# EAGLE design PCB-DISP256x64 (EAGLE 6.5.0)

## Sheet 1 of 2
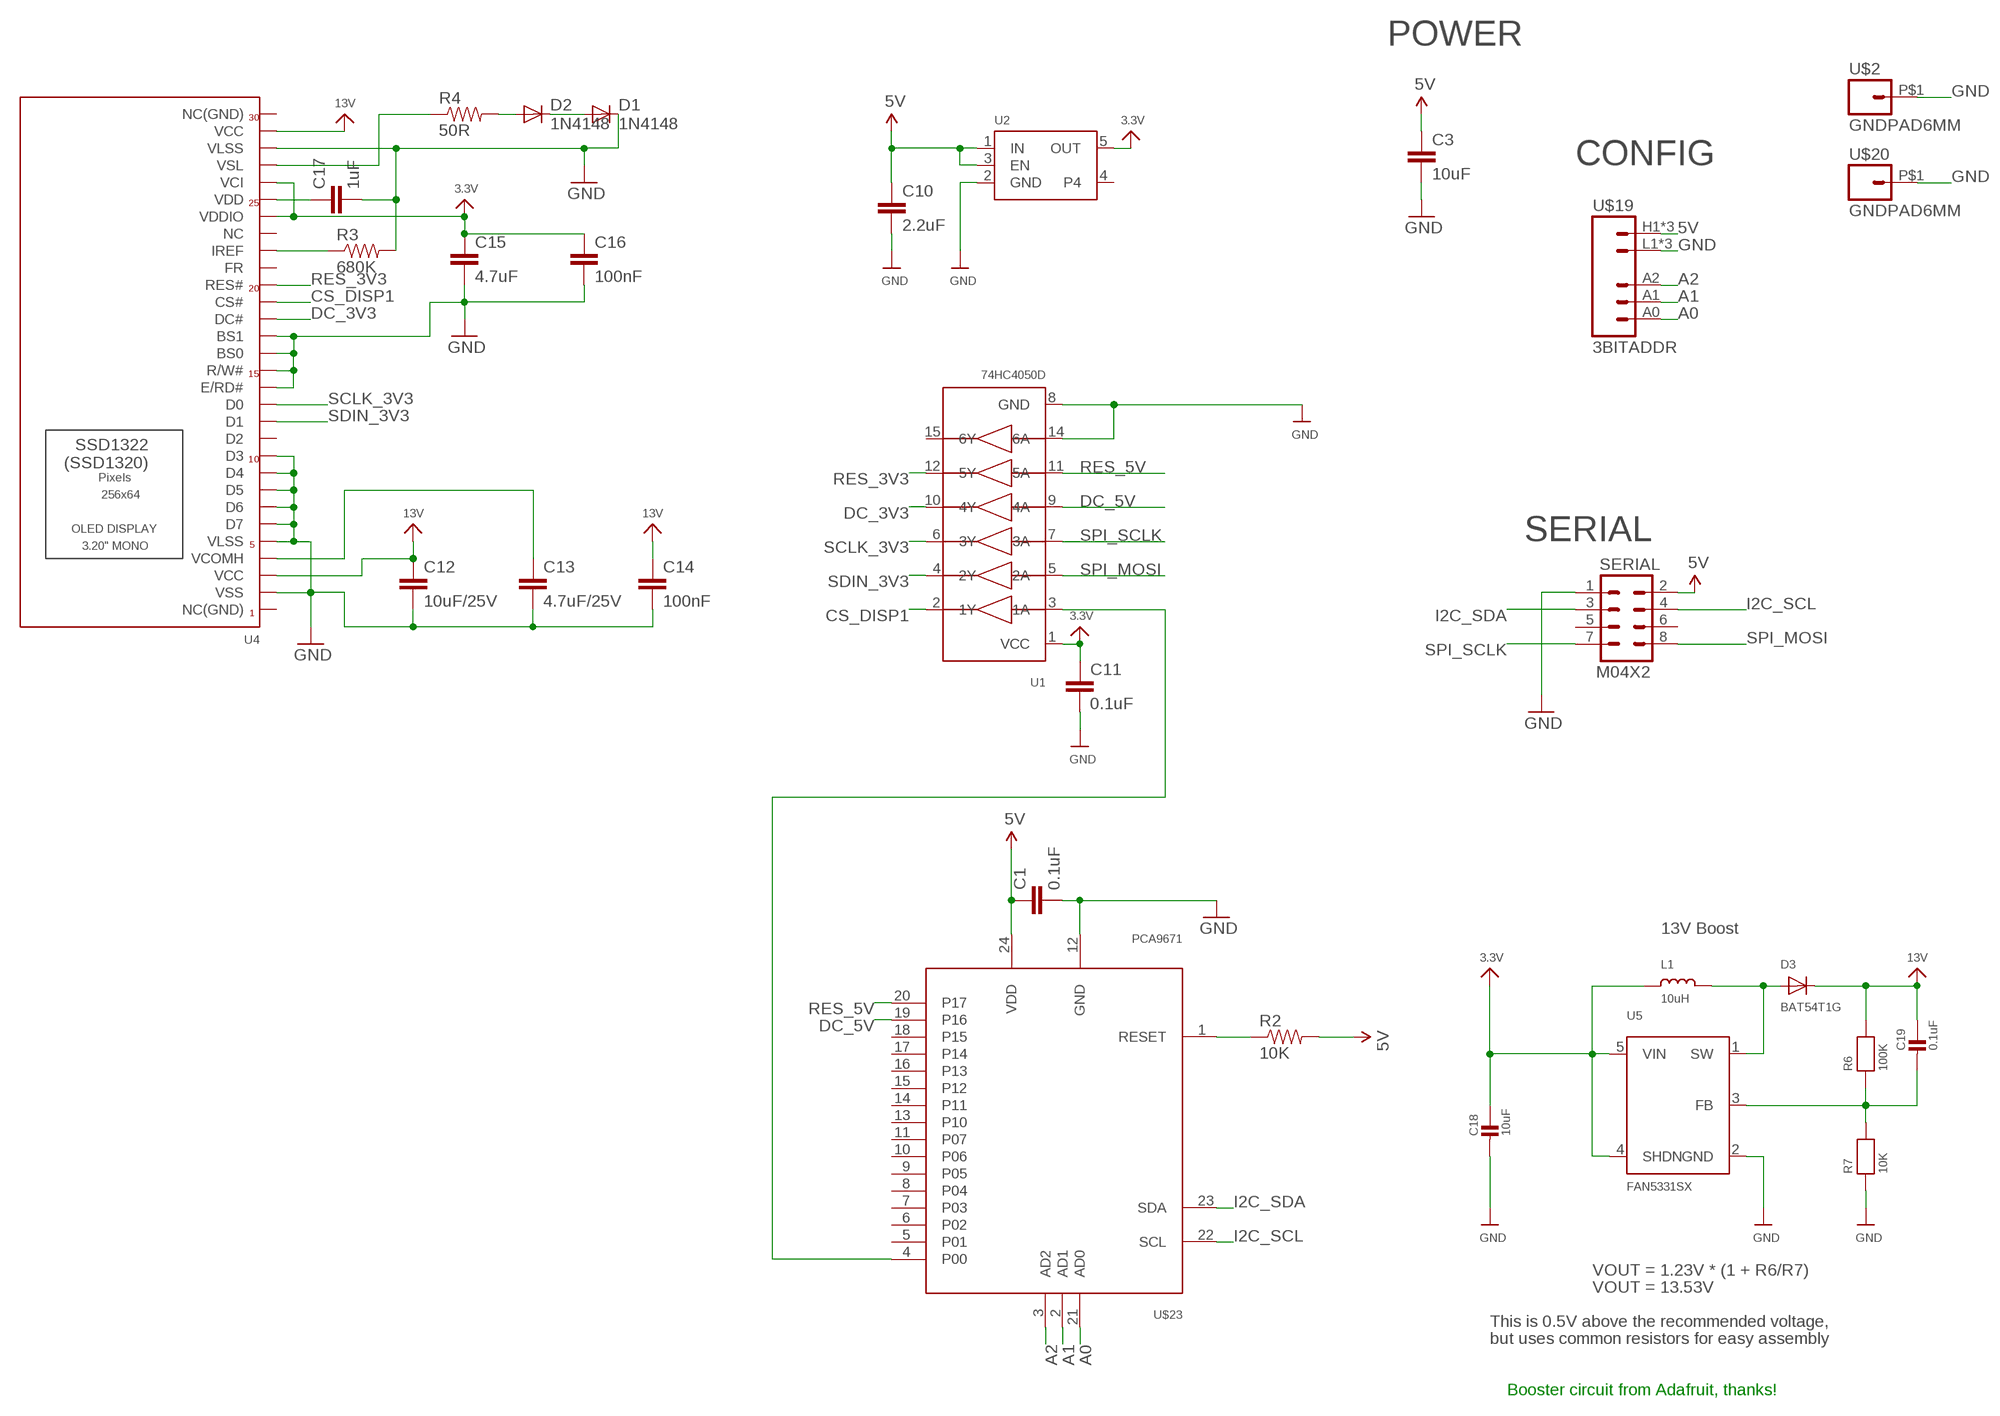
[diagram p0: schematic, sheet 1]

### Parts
C1  0.1uF  CAP0603-CAP  [0603-CAP]
C3  10uF  CAP0805  [0805]
C10  2.2uF  CAP0603-CAP  [0603-CAP]
C11  0.1uF  CAP0603-CAP  [0603-CAP]
C12  10uF/25V  CAP0805  [0805]
C13  4.7uF/25V  CAP0805  [0805]
C14  100nF  CAP0603-CAP  [0603-CAP]
C15  4.7uF  CAP0805  [0805]
C16  100nF  CAP0603-CAP  [0603-CAP]
C17  1uF  CAP0603-CAP  [0603-CAP]
C18  10uF  CAP_CERAMIC0805  [0805]
C19  0.1uF  CAP_CERAMIC0805  [0805]
D1  1N4148  DIODESOD  [SOD-323]
D2  1N4148  DIODESOD  [SOD-323]
D3  BAT54T1G  DIODESOD-123  [SOD-123]
L1  10uH  INDUCTOR  [INDUCTOR_1007]
R2  10K  RESISTOR0603-RES  [0603-RES]
R3  680K  RESISTOR0603-RES  [0603-RES]
R4  50R  RESISTOR0603-RES  [0603-RES]
R6  100K  RESISTOR0805  [0805]
R7  10K  RESISTOR0805  [0805]
SERIAL  M04X2  [2X4]
U1  74HC4050D  [SOIC16]
U2  VREG_SOT23-5  [SOT23-5]
U4  ER_OLED032-1TOP  [FPC_XF2M-3015-1A]
U5  FAN5331SX  FAN5331  [SOT23-5@1]
U$2  GNDPAD6MM  [3.2MMPAD6MM]
U$19  3BITADDR  [3BITADDR]
U$20  GNDPAD6MM  [3.2MMPAD6MM]
U$23  PCA9671  [TSSOP24]

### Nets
3.3V [Power]: C11.1 C15.1 C16.1 C18.1 L1.P$1 U1.1(VCC) U2.5(OUT) U4.P$5(VCI) U4.P$7(VDDIO) U5.4(SHDN) U5.5(VIN)
5V [Power]: C1.1 C3.1 C10.1 R2.2 SERIAL.2 U2.1(IN) U2.3(EN) U$19.H1(VCC) U$19.H2(VCC) U$19.H3(VCC) U$23.24(VDD)
13V [Power]: C12.1 C14.1 C19.1 D3.C R6.2 U4.P$2(VCC) U4.P$28(VCC)
A0: U$19.A0 U$23.21(AD0)
A1: U$19.A1 U$23.2(AD1)
A2: U$19.A2 U$23.3(AD2)
CS_DISP1: U1.2(1Y) U4.P$12(CS#)
DC_3V3: U1.10(4Y) U4.P$13(DC#)
DC_5V: U1.9(4A) U$23.19(P16)
GND [Power]: C1.2 C3.2 C10.2 C11.2 C12.2 C13.2 C14.2 C15.2 C16.2 C17.2 C18.2 D1.1(C) R3.2 R7.1 SERIAL.1 U1.8(GND) U1.14(6A) U2.2(GND) U4.P$3(VLSS) U4.P$14(BS1) U4.P$15(BS0) U4.P$16(R/W#) U4.P$17(E/RD#) U4.P$21(D3) U4.P$22(D4) U4.P$23(D5) U4.P$24(D6) U4.P$25(D7) U4.P$26(VLSS) U4.P$29(VSS) U5.2(GND) U$2.P$1 U$19.L1(GND) U$19.L2(GND) U$19.L3(GND) U$20.P$1 U$23.12(GND)
I2C_SCL: SERIAL.4 U$23.22(SCL)
I2C_SDA: SERIAL.3 U$23.23(SDA)
N$1: R2.1 U$23.1(RESET)
N$3: U1.3(1A) U$23.4(P00)
N$5: C13.1 U4.P$27(VCOMH)
N$6: R4.1 U4.P$4(VSL)
N$10: R3.1 U4.P$9(IREF)
N$11: D2.2(A) R4.2
N$12: C17.1 U4.P$6(VDD)
N$13: D1.2(A) D2.1(C)
N$14: D3.A L1.P$2 U5.1(SW)
N$15: C19.2 R6.1 R7.2 U5.3(FB)
RES_3V3: U1.12(5Y) U4.P$11(RES#)
RES_5V: U1.11(5A) U$23.20(P17)
SCLK_3V3: U1.6(3Y) U4.P$18(D0)
SDIN_3V3: U1.4(2Y) U4.P$19(D1)
SPI_MOSI: SERIAL.8 U1.5(2A)
SPI_SCLK: SERIAL.7 U1.7(3A)
Unconnected: SERIAL.5 SERIAL.6 U1.15(6Y) U2.4 U4.P$1(NC(GND)) U4.P$8(NC) U4.P$10(FR) U4.P$20(D2) U4.P$30(NC(GND)) U$23.5(P01) U$23.6(P02) U$23.7(P03) U$23.8(P04) U$23.9(P05) U$23.10(P06) U$23.11(P07) U$23.13(P10) U$23.14(P11) U$23.15(P12) U$23.16(P13) U$23.17(P14) U$23.18(P15)

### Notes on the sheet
- POWER
- CONFIG
- SERIAL
- 13V Boost
- VOUT = 1.23V * (1 + R6/R7)
- VOUT = 13.53V
- This is 0.5V above the recommended voltage,
- but uses common resistors for easy assembly
- Booster circuit from Adafruit, thanks!

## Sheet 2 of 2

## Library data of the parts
C1 C3 C10-C17 = SparkFun:CAP: Capacitor
C18 C19 = microbuilder:CAP_CERAMIC: Ceramic Capacitors
D1 D2 = SparkFun:DIODE: Diode
D3 = microbuilder:DIODE: Diode
L1 = microbuilder:INDUCTOR: Inductors
R2-R4 = SparkFun:RESISTOR: Resistor
R6 R7 = microbuilder:RESISTOR: Resistors
SERIAL = SparkFun:M04X2
U1 = microbuilder:74HC4050D: 6-channel level shifter 74HC4050D - 2V-6V Supply Digikey: 74HC4050D,653-ND Mouser: 771-74HC4050D-T
U2 = microbuilder:VREG_SOT23-5: SOT23-5 Fixed Voltage Regulators To better organise some of the SOT23-5 fixed voltage regulators in this library, this new part was created. Part Current Out V Out V In V Dropout Digikey Part No. ADP121 150mA 3.3V 3.4-5.5V 0.09V @ 150mA ADP121-AUJZ33R7CT-ND ADP121 150mA 3.0V 3.1-5.5V 0.09V @ 150mA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
U4 = SKAARHOJ:ER_OLED032-1: 128x128 1.5" RGB OLED - UG-2828GDEDF11 30-Pin 0.5mm Pitch FPC Cable (Top+Bottom Contacts) - OMRON XF2M-3015-1A (Digikey: OR723TR-ND) This FPC connector has contacts on the top and bottom, but the appropriate pin needs to be selected depending on whether the OLED will be inserted right-side up (use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
U5 = microbuilder:FAN5331: FAN5331 - LED/OLED 20V Boost Converter Digikey: FAN5331SXCT-ND
U$2 U$20 = SKAARHOJ:GNDPAD
U$19 = SKAARHOJ:3BITADDR
U$23 = SKAARHOJ:PCA9671

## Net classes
0 default: width 0.203 mm, drill 0.406 mm, clearance 0.152 mm
1 Power: width 0.203 mm, drill 0.61 mm, clearance 0.152 mm
3 INput lines: width 0.203 mm, drill 0.406 mm, clearance 0.152 mm

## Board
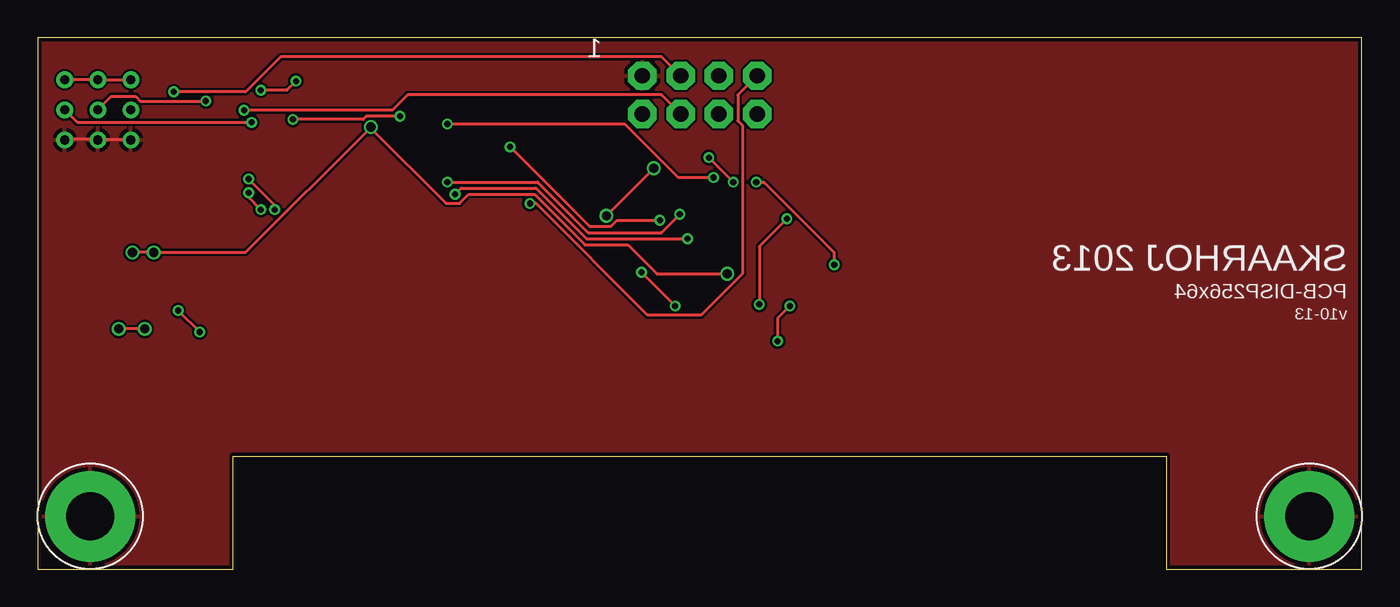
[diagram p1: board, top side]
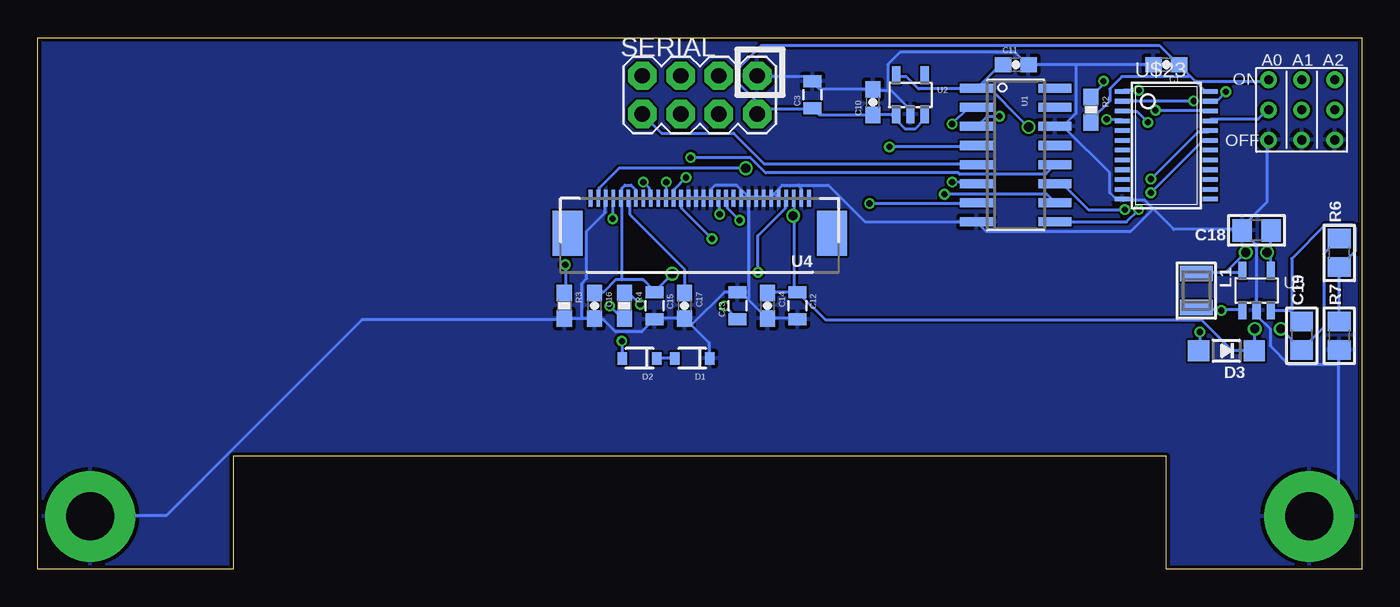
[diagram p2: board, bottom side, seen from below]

Size 88 x 35.3 mm. Coordinates in mm from the lower left corner, seen from the top.
Outline: 88,0 88,35.3 0,35.3 0,0 13,0 13,7.5 75,7.5 75,0 88,0
Copper layers (1*16): Top 0.035mm / dielectric 1.5mm / Bottom 0.035mm
Design rules "Fusion_eagle_rule_v1.1": minimum track width 6mil, minimum drill 12mil, track to track 6mil, track to pad 6mil, pad to pad 6mil, via to via 6mil, smd to smd 0mil, copper to edge 10mil, drill to drill 10mil, minimum pad ring 10mil, minimum via ring 6mil, stop-mask expansion 2mil, vias tented up to drill 100mil, thermal gap 10mil

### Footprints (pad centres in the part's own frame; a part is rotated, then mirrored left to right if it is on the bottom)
0603-CAP = smd 1.1 x 1: 1 -0.85,0; 2 0.85,0
0805 = smd 0.8 x 1.2: 1 -0.9,0; 2 0.9,0
0805' = smd 1.3 x 1.5: 1 -0.95,0; 2 0.95,0
SOD-323 = smd 0.63 x 0.83: 1 -1.15,0; 2 1.15,0
SOD-123 = smd 1.4 x 1.4: A 1.85,0; C -1.85,0
INDUCTOR_1007 = smd 1.016 x 2.2: P$1 -1.127,0; P$2 1.127,0
0603-RES = smd 1.1 x 1: 1 -0.85,0; 2 0.85,0
2X4 = drill 1.016 pad 1.88 octagon: 1 -3.81,-1.27; 2 -3.81,1.27; 3 -1.27,-1.27; 4 -1.27,1.27; 5 1.27,-1.27; 6 1.27,1.27; 7 3.81,-1.27; 8 3.81,1.27
SOIC16 = smd 0.6 x 2.2: 1 -4.445,-2.6; 2 -3.175,-2.6; 3 -1.905,-2.6; 4 -0.635,-2.6; 5 0.635,-2.6; 6 1.905,-2.6; 7 3.175,-2.6; 8 4.445,-2.6; 9 4.445,2.6; 10 3.175,2.6; 11 1.905,2.6; 12 0.635,2.6; 13 -0.635,2.6; 14 -1.905,2.6; 15 -3.175,2.6; 16 -4.445,2.6
SOT23-5 = smd 0.55 x 1.2: 1 -0.95,-1.3; 2 0,-1.3; 3 0.95,-1.3; 4 0.95,1.3; 5 -0.95,1.3
FPC_XF2M-3015-1A = smd 0.25 x 1.1: P$1 7.25,-2.63; P$2 6.75,-2.63; P$3 6.25,-2.63; P$4 5.75,-2.63; P$5 5.25,-2.63; P$6 4.75,-2.63; P$7 4.25,-2.63; P$8 3.75,-2.63; P$9 3.25,-2.63; P$10 2.75,-2.63; P$11 2.25,-2.63; P$12 1.75,-2.63; P$13 1.25,-2.63; P$14 0.75,-2.63; P$15 0.25,-2.63; P$16 -0.25,-2.63; P$17 -0.75,-2.63; P$18 -1.25,-2.63; P$19 -1.75,-2.63; P$20 -2.25,-2.63; P$21 -2.75,-2.63; P$22 -3.25,-2.63; P$23 -3.75,-2.63; P$24 -4.25,-2.63; P$25 -4.75,-2.63; P$26 -5.25,-2.63; P$27 -5.75,-2.63; P$28 -6.25,-2.63; P$29 -6.75,-2.63; P$30 -7.25,-2.63 | smd 2 x 3: SUPPORT1 8.79,-0.305; SUPPORT2 -8.79,-0.305
SOT23-5@1 = smd 0.55 x 1.2: 1 -0.95,-1.3; 2 0,-1.3; 3 0.95,-1.3; 4 0.95,1.3; 5 -0.95,1.3
3.2MMPAD6MM = drill 3.2 pad 6: P$1 0,0
3BITADDR = drill 0.6: A0 -2.2,0; A1 0,0; A2 2.2,0; H1 -2.2,2; H2 0,2; H3 2.2,2; L1 -2.2,-2; L2 0,-2; L3 2.2,-2
TSSOP24 = smd 0.305 x 0.991: 1 -4.225,-2.918; 2 -3.575,-2.918; 3 -2.925,-2.918; 4 -2.275,-2.918; 5 -1.625,-2.918; 6 -0.975,-2.918; 7 -0.325,-2.918; 8 0.325,-2.918; 9 0.975,-2.918; 10 1.625,-2.918; 11 2.275,-2.918; 12 2.925,-2.918; 13 2.925,2.918; 14 2.275,2.918; 15 1.625,2.918; 16 0.975,2.918; 17 0.325,2.918; 18 -0.325,2.918; 19 -0.975,2.918; 20 -1.625,2.918; 21 -2.275,2.918; 22 -2.925,2.918; 23 -3.575,2.918; 24 -4.225,2.918

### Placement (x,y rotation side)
C1  13,33.5 180 bottom
C3  36.5,31.5 90 bottom
C10  32.5,31 90 bottom
C11  23,33.5 0 bottom
C12  37.5,17.5 270 bottom
C13  41.5,17.5 90 bottom
C14  39.5,17.5 270 bottom
C15  47,17.5 270 bottom
C16  51,17.5 270 bottom
C17  45,17.5 270 bottom
C18  10uF  [0805']  7,22.5 180 bottom
C19  0.1uF  [0805']  4,15.5 90 bottom
D1  44.5,14 180 bottom
D2  48,14 180 bottom
D3  9,14.5 180 bottom
L1  11,18.5 270 bottom
R2  18,30.5 270 bottom
R3  53,17.5 270 bottom
R4  49,17.5 270 bottom
R6  100K  [0805']  1.5,21 90 bottom
R7  10K  [0805']  1.5,15.5 90 bottom
SERIAL  44,31.5 180 bottom
U1  23,27.5 270 bottom
U2  30,31.5 0 bottom
U4  44,22 180 bottom
U5  7,18.5 0 bottom
U$2  3.5,3.5 0 top
U$19  4,30.5 0 bottom
U$20  84.5,3.5 0 top
U$23  13,27.5 270 bottom

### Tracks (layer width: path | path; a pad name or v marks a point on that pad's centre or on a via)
3.3V  (via drill 0.61)
  Top 0.203: v6.3,21.03 v7.72,21.03 13.82,21.03 v22.15,29.36 22.15,29.26 27.13,24.28 28.04,24.28 28.65,24.89 33.02,24.89 36.37,21.54 39.22,21.54 41.15,19.61 v45.82,19.61
  Bottom 0.203: U4.P$7 48.26,24.69 48.26,25.2 48.56,25.5 48.97,25.5 49.17,25.3 49.17,24.69 U4.P$5 49.17,24.59 49.17,19.2 | 49.17,19.2 47.75,19.2 47.04,18.49 C15.1 46.94,18.49 v45.82,19.61 | 49.17,19.2 49.58,19.2 50.39,18.39 50.9,18.39 C16.1 | 25.15,32.36 25.5,32 U1.1 25.6,31.9 29.46,31.9 30.28,32.72 30.89,32.72 U2.5 | 25.15,32.36 24.08,33.43 23.88,33.43 C11.1 | 6.1,21.03 6.1,22.45 C18.1 | 6.1,21.03 6.1,19.81 U5.4 | 9.04,19.71 10.97,19.71 L1.P$1 | 9.04,19.71 8.03,19.71 U5.5 | v6.3,21.03 6.1,21.03 | 9.04,19.71 v7.72,21.03 | v22.15,29.36 25.15,32.36
5V
  Top 0.203: U$19.H3 1.83,32.51 3.96,32.51 U$19.H2 4.06,32.51 6.2,32.51 U$19.H1
  Bottom 0.203: 31.29,30.18 30.99,30.18 U2.1 | 31.29,30.18 32.41,30.18 C10.1 32.51,30.18 36.07,30.18 36.47,30.58 C3.1 36.58,30.58 39.83,30.58 40.13,30.28 SERIAL.2 39.93,30.58 39.93,30.79 41.45,32.31 41.45,33.22 39.93,34.75 13.41,34.75 12.19,33.53 C1.1 12.09,33.43 11.43,32.77 | 31.29,30.18 30.38,29.26 29.67,29.26 29.06,29.87 29.06,30.18 U2.3 | 11.43,32.77 11.02,32.36 | 11.02,32.36 10.46,31.8 10.16,31.8 U$23.24 | R2.2 17.98,29.67 17.98,29.87 16.76,31.09 16.76,31.9 15.95,32.72 11.48,32.72 11.43,32.77 | U$19.H1 6.3,32.41 10.97,32.41 11.02,32.36
13V  (via drill 0.61)
  Top 0.203: v37.8,23.47 v40.95,26.62 | v7.11,15.95 v5.38,15.95
  Bottom 0.203: R6.2 1.52,21.95 2.54,20.93 2.54,16.05 3.96,14.63 C19.1 4.06,14.63 v5.38,15.95 | 37.69,23.47 37.69,18.59 37.59,18.49 C12.1 | 37.69,23.47 37.69,24.59 U4.P$28 | C14.1 39.42,18.39 37.59,18.39 C12.1 | v40.95,26.62 49.38,26.62 50.7,25.3 50.7,24.69 U4.P$2 | 37.69,23.47 v37.8,23.47 | C12.1 35.66,16.56 10.67,16.56 8.64,14.53 7.21,14.53 D3.C 7.11,14.53 v7.11,15.95
A0
  Bottom 0.203: U$23.21 10.06,29.87 6.91,29.87 6.3,30.48 U$19.A0
A1  (via drill 0.41)
  Top 0.203: v11.18,31.09 6.81,31.09 6.5,31.39 4.88,31.39 4.06,30.58 U$19.A1
  Bottom 0.203: v11.18,31.09 15.85,31.09 U$23.2
A2  (via drill 0.41)
  Top 0.203: v14.22,29.67 2.64,29.67 1.83,30.48 U$19.A2
  Bottom 0.203: v14.22,29.67 14.94,30.38 15.85,30.38 U$23.3
CS_DISP1  (via drill 0.41)
  Top 0.203: v44.91,26.01 42.57,26.01 39.01,29.57 v27.23,29.57
  Bottom 0.203: v44.91,26.01 45.72,25.2 45.72,24.69 U4.P$12 | v27.23,29.57 26.21,30.58 25.6,30.58 U1.2
DC_3V3  (via drill 0.41)
  Top 0.203: v43.18,21.95 36.47,21.95 33.12,25.3 28.14,25.3 v27.74,24.89
  Bottom 0.203: v43.18,21.95 45.21,23.98 45.21,24.59 U4.P$13 | v27.74,24.89 20.93,24.89 20.42,24.38 U1.10
DC_5V  (via drill 0.41)
  Top 0.203: v14.02,24.99 14.02,24.69 v14.83,23.88
  Bottom 0.203: v14.02,24.99 10.57,28.45 10.16,28.45 U$23.19 | v14.83,23.88 15.65,23.06 20.32,23.06 U1.9
GND
  Top 0.203: U$19.L3 1.83,28.55 3.96,28.55 U$19.L2 4.06,28.55 6.2,28.55 U$19.L1
  Bottom 0.203: 1.52,13.61 1.52,5.49 3.45,3.56 U$2.P$1 | 1.52,13.61 1.52,14.53 R7.1 | 31.5,31.8 32.41,31.8 C10.2 32.51,31.9 36.07,31.9 36.47,32.31 C3.2 36.58,32.41 36.88,32.72 40.13,32.72 SERIAL.1 | 31.5,31.8 31.29,31.8 30.07,30.58 30.07,30.28 U2.2 | 19,33.53 22.15,33.53 C11.2 22.25,33.53 23.06,34.34 30.68,34.34 31.5,33.53 31.5,31.8 | 19,33.53 13.92,33.53 C1.2 | 19,33.53 19,30.28 19.81,29.46 20.32,29.46 U1.14 19.71,29.46 19.71,29.26 16.76,26.31 16.76,24.99 16.36,24.59 15.95,24.59 U$23.12 15.85,24.49 14.43,24.49 13.87,23.93 | 13.87,23.93 12.5,22.55 8.03,22.55 C18.2 | C18.2 7.92,22.45 7.01,21.54 7.01,17.27 U5.2 6.91,17.17 6.91,16.76 6.1,15.95 6.1,14.83 4.88,13.61 1.52,13.61 | U$19.L1 6.3,28.45 6.3,24.38 8.03,22.66 C18.2 | U4.P$14 44.7,24.69 44.3,24.69 U4.P$15 44.2,24.69 43.79,24.69 U4.P$16 43.69,24.69 43.28,24.69 U4.P$17 43.28,24.79 43.28,25.2 42.98,25.5 41.55,25.5 40.84,24.79 U4.P$22 | 37.44,25.45 37.49,25.5 38.51,25.5 39.06,24.94 | 37.44,25.45 37.29,25.3 37.29,24.69 U4.P$29 | 39.32,24.69 39.06,24.94 | 39.32,24.69 U4.P$25 | 39.06,24.94 38.81,24.69 U4.P$26 | 39.32,24.69 39.73,24.69 U4.P$24 39.83,24.69 40.23,24.69 U4.P$23 40.34,24.69 40.74,24.69 U4.P$22 | U4.P$21 41.25,24.69 40.84,24.69 U4.P$22 | 37.44,25.45 37.39,25.5 35.46,25.5 33.02,23.06 25.6,23.06 U1.8 25.5,22.96 24.99,22.45 15.34,22.45 13.87,23.93 | 51.82,16.66 52.93,16.66 R3.2 53.03,16.56 66.45,16.56 79.45,3.56 84.43,3.56 U$20.P$1 | 51.82,16.66 51,16.66 C16.2 50.9,16.56 50.39,16.56 49.58,15.75 47.85,15.75 47.04,16.56 C15.2 46.94,16.66 45.01,16.66 C17.2 | 51.82,16.66 51.82,19 51.51,19.3 51.51,22.45 50.29,23.67 50.29,24.59 U4.P$3
  Bottom 0.203: D1.1 43.38,14.02 43.38,15.04 44.91,16.56 C17.2 | C12.2 37.59,16.66 39.42,16.66 C14.2 39.52,16.66 40.79,17.93 | 40.79,17.93 41.25,18.39 41.45,18.39 C13.2 41.55,18.39 42.37,18.39 44.5,16.26 C17.2 | U4.P$22 40.74,24.59 40.74,17.98 40.79,17.93
  pour Top: 0,0 88,0 88,35.5 0,35.5
  pour Bottom: 0,0 88,0 88,35.5 0,35.5
I2C_SCL  (via drill 0.41)
  Top 0.203: v13.72,30.48 23.57,30.48 24.59,31.5 41.45,31.5 42.67,30.28 SERIAL.4
  Bottom 0.203: v13.72,30.48 10.16,30.48 U$23.22
I2C_SDA  (via drill 0.41)
  Top 0.203: v9.04,31.7 13.82,31.7 16.15,34.04 41.45,34.04 42.67,32.82 SERIAL.3
  Bottom 0.203: v9.04,31.7 9.65,31.09 10.06,31.09 U$23.23
N$1  (via drill 0.41)
  Top 0.203: v14.83,31.8 16.56,31.8 v17.17,32.41
  Bottom 0.203: v14.83,31.8 15.85,31.8 U$23.1 | v17.17,32.41 17.17,32.21 17.98,31.39 R2.1
N$3  (via drill 0.41)
  Top 0.203: v16.97,29.87 21.64,29.87 21.84,30.07 v24.08,30.07
  Bottom 0.203: v16.97,29.87 15.95,29.87 U$23.4 | v24.08,30.07 24.89,30.07 25.5,29.46 U1.3
N$5  (via drill 0.41)
  Top 0.203: v42.37,17.48 v40.13,19.71
  Bottom 0.203: v40.13,19.71 40.13,22.15 38.3,23.98 38.3,24.59 U4.P$27 | v42.37,17.48 41.55,16.66 C13.1
N$6  (via drill 0.41)
  Top 0.203: v47.95,17.58 47.95,21.44 v49.78,23.27
  Bottom 0.203: v47.95,17.58 48.67,18.29 48.97,18.29 R4.1 | v49.78,23.27 49.78,24.59 U4.P$4
N$10  (via drill 0.41)
  Top 0.203: v52.93,20.22 52.93,21.03 48.26,25.7 v47.75,25.7
  Bottom 0.203: v52.93,20.22 52.93,18.39 R3.1 | v47.75,25.7 47.35,25.3 47.35,24.69 U4.P$9
N$11  (via drill 0.41)
  Top 0.203: v49.17,15.14 49.17,16.66 v49.99,17.48
  Bottom 0.203: v49.17,15.14 49.17,14.02 D2.2 | v49.99,17.48 49.07,16.56 R4.2
N$12
  Bottom 0.203: C17.1 45.01,18.39 45.01,19.91 48.67,23.57 48.67,24.59 U4.P$6
N$13
  Bottom 0.203: D1.2 45.72,14.02 46.84,14.02 D2.1
N$14  (via drill 0.41)
  Top 0.203: v9.35,17.17 v10.77,15.75
  Bottom 0.203: 9.35,17.27 10.97,17.27 L1.P$2 | 9.35,17.27 8.03,17.27 U5.1 | v10.77,15.75 10.77,14.53 D3.A | 9.35,17.27 v9.35,17.17
N$15
  Bottom 0.203: 4.72,17.12 4.06,16.46 C19.2 | 4.72,17.12 4.78,17.17 5.99,17.17 U5.3 | R7.2 1.52,16.46 1.52,20.02 R6.1 1.42,20.12 0.41,21.13 0.41,22.66 0.61,22.86 2.44,22.86 4.67,20.62 4.67,17.17 4.72,17.12
RES_3V3  (via drill 0.41)
  Top 0.203: v44.6,27.33 v46.23,25.7
  Bottom 0.203: v46.23,25.7 46.23,24.69 U4.P$11 | v44.6,27.33 40.64,27.33 39.62,26.31 26.82,26.31 26.72,26.21 21.03,26.21 20.42,26.82 U1.12
RES_5V  (via drill 0.41)
  Top 0.203: v14.02,25.91 15.75,24.18 v15.75,23.88
  Bottom 0.203: v14.02,25.91 10.87,29.06 10.16,29.06 U$23.20 | v15.75,23.88 18.19,23.88 19.81,25.5 20.32,25.5 U1.11
SCLK_3V3  (via drill 0.41)
  Top 0.203: v42.67,23.57 41.45,22.35 36.58,22.35 33.22,25.7 v27.23,25.7
  Bottom 0.203: v42.67,23.57 42.67,24.59 U4.P$18 | v27.23,25.7 25.7,25.7 25.6,25.6 U1.6
SDIN_3V3  (via drill 0.41)
  Top 0.203: v41.35,23.16 38.51,23.16 38.1,22.76 36.68,22.76 v31.39,28.04
  Bottom 0.203: v41.35,23.16 42.16,23.98 42.16,24.59 U4.P$19 | v31.39,28.04 25.6,28.04 U1.4
SPI_MOSI
  Bottom 0.203: U1.5 25.6,26.92 39.73,26.92 41.76,28.96 46.53,28.96 47.75,30.18 SERIAL.8
SPI_SCLK  (via drill 0.41)
  Top 0.203: v32.72,24.28 33.12,24.28 40.54,16.87 44.09,16.87 46.84,19.61 46.84,29.46 46.53,29.77 46.53,31.5 47.75,32.72 SERIAL.7
  Bottom 0.203: v32.72,24.28 25.6,24.28 U1.7

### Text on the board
_tsilk: 1 | SKAARHOJ 2013 | PCB-DISP256x64 | v10-13

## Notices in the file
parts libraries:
SparkFun: Licensing: CC v3.0 Share-Alike You are welcome to use this library for commercial purposes.
